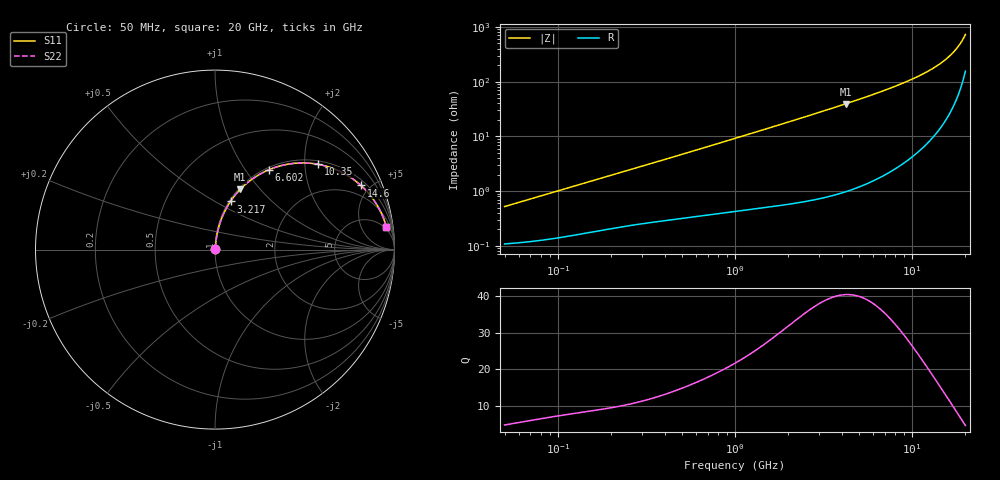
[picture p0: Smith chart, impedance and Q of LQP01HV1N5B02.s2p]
!Murata Part Number: LQP01HV1N5B02
!These Parameters are Measured in Series Mode Connection
!  o--[Z]--o
!Port1  Port2
!  o-------o
!Freq. Start=50[MHz] Stop=20[GHz], 401[Steps]
# Hz S RI R 50
!Freq.(Hz) S11(Real) S11(Imag) S21(Real) S21(Imag) S12(Real) S12(Imag) S22(Real) S22(Imag)
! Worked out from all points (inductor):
!   401 points, 50 MHz to 20 GHz, reference 50 ohm
!   read as one part in series: L = 1.62 nH near 51.52 MHz
!   highest Q = 40.5 at 4.212 GHz (marker M1), where L = 1.49 nH
!   S11 on the Smith chart (normalised r, x): 50 MHz: 1.00, +0.01; 3.217 GHz: 1.02, +0.59; 6.602 GHz: 1.04, +1.30; 10.35 GHz: 1.09, +2.34; 14.6 GHz: 1.30, +4.40; 20 GHz: 4, +14
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5e7  0.00111 0.00508  0.9989 -0.00508  0.9989 -0.00508  0.00111 0.00508
1.364002e8  0.00183 0.0135  0.9982 -0.0135  0.9982 -0.0135  0.00183 0.0135
3.721004e8  0.004 0.0348  0.996 -0.0348  0.996 -0.0348  0.004 0.0348
6.380365e8  0.00693 0.0585  0.9931 -0.0585  0.9931 -0.0585  0.00693 0.0585
1e9  0.0125 0.0902  0.9875 -0.0902  0.9875 -0.0902  0.0125 0.0902
1.689197e9  0.0281 0.1491  0.9719 -0.1491  0.9719 -0.1491  0.0281 0.1491
2.728004e9  0.0645 0.2324  0.9355 -0.2324  0.9355 -0.2324  0.0645 0.2324
3.216634e9  0.0865 0.2686  0.9135 -0.2686  0.9135 -0.2686  0.0865 0.2686
4.212059e9  0.14 0.3349  0.86 -0.3349  0.86 -0.3349  0.14 0.3349
5.273168e9  0.2072 0.3929  0.7928 -0.3929  0.7928 -0.3929  0.2072 0.3929
6.601595e9  0.3011 0.4453  0.6989 -0.4453  0.6989 -0.4453  0.3011 0.4453
7.442007e9  0.3634 0.4666  0.6366 -0.4666  0.6366 -0.4666  0.3634 0.4666
8.907419e9  0.4724 0.4827  0.5276 -0.4827  0.5276 -0.4827  0.4724 0.4827
1.034674e10  0.5746 0.4752  0.4254 -0.4752  0.4254 -0.4752  0.5746 0.4752
1.238412e10  0.7027 0.4328  0.2973 -0.4328  0.2973 -0.4328  0.7027 0.4328
1.354865e10  0.7648 0.396  0.2352 -0.396  0.2352 -0.396  0.7648 0.396
1.460232e10  0.8134 0.3573  0.1866 -0.3573  0.1866 -0.3573  0.8134 0.3573
1.597544e10  0.8659 0.3013  0.1341 -0.3013  0.1341 -0.3013  0.8659 0.3013
1.721783e10  0.9032 0.2475  0.0968 -0.2475  0.0968 -0.2475  0.9032 0.2475
1.828096e10  0.928 0.2004  0.072 -0.2004  0.072 -0.2004  0.928 0.2004
1.940974e10  0.9477 0.1503  0.0523 -0.1503  0.0523 -0.1503  0.9477 0.1503
2e10  0.9554 0.1244  0.0446 -0.1244  0.0446 -0.1244  0.9554 0.1244
